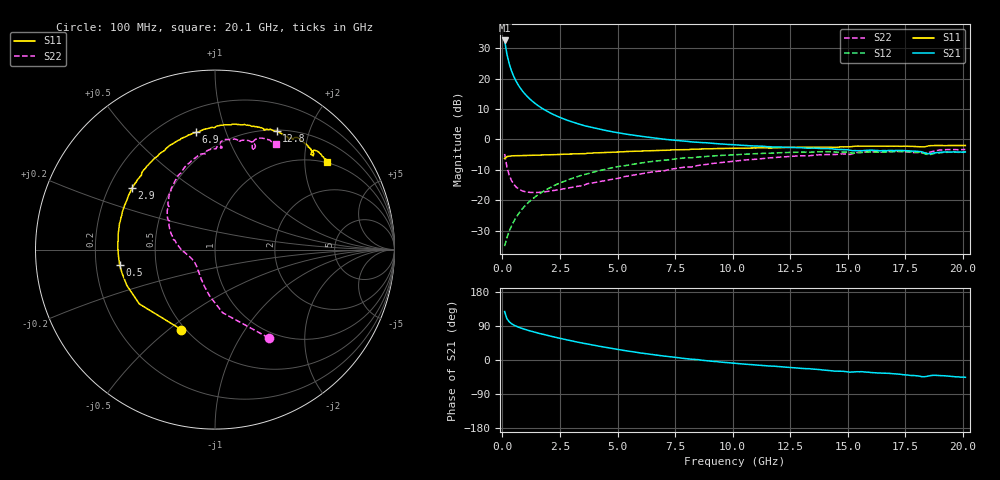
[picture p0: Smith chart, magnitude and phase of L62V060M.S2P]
!  Infineon Technologies AG
! BFR380L3 , PF131585-7, No.6, Th 09.10.01, soldered on pcb-board, measured with PP GSG850
!  Vce=2.0 V,  Ic=60.0 mA
! Common Emitter S-Parameters:  15. November 2001
#  GHz  S  MA  R  50
! f  S11  S21  S12  S22
! GHz  Mag  Ang  Mag  Ang  Mag  Ang  Mag  Ang
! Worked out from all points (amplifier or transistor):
!   201 points, 100 MHz to 20.1 GHz, reference 50 ohm
!   highest |S21| = 32.6 dB at 100 MHz (marker M1)
!   |S21| within 3 dB of that: start of sweep to 166.2 MHz
!   unconditionally stable (mu >= 1): 730.2 MHz to 4.314 GHz; 18.27 GHz to 18.57 GHz
!   at 3.4 GHz: K = 1.02, MAG = 7.5 dB, |S12| = -11.9 dB
!   at 10.1 GHz: K = 0.96, MSG = 1.6 dB, |S12| = -5.0 dB
!   at 20.1 GHz: K = 0.99, MSG = 0.0 dB, |S12| = -4.2 dB
!   S11 on the Smith chart (normalised r, x): 100 MHz: 0.48, -0.55; 500 MHz: 0.30, -0.07; 2.9 GHz: 0.30, +0.30; 6.9 GHz: 0.34, +0.79; 12.8 GHz: 0.52, +1.52; 20.1 GHz: 0.97, +2.58
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0.1  0.4834 -112.8  42.61 127.7  0.01746 57.2  0.5762 -58.6
0.2  0.519 -144.3  25.29 109.1  0.02393 58.7  0.3544 -83.1
0.3  0.5302 -157.8  17.6 100.9  0.03099 61.3  0.2588 -96.8
0.4  0.534 -165.7  13.42 95.8  0.0376 64.7  0.2098 -106.9
0.5  0.5382 -170.9  10.82 92.1  0.04477 67.0  0.1822 -114.7
0.6  0.5385 -175.0  9.05 89.3  0.05207 68.5  0.1646 -121.2
0.7  0.5399 -178.2  7.796 86.7  0.0592 69.4  0.1535 -126.7
0.8  0.541 178.9  6.84 84.4  0.06676 70.0  0.1459 -131.3
1  0.5426 174.1  5.506 80.4  0.08169 70.6  0.1375 -138.7
1.2  0.5468 169.9  4.609 76.8  0.0965 70.2  0.1343 -144.4
1.5  0.5516 164.6  3.717 71.9  0.119 69.2  0.1336 -151.0
1.8  0.5535 159.6  3.123 67.2  0.1412 67.9  0.1364 -156.3
2.9  0.5761 143.5  2.018 51.9  0.2196 60.9  0.1594 -170.7
3.5  0.583 135.3  1.711 44.3  0.2611 56.5  0.1739 -176.1
5.1  0.6197 116.9  1.27 26.8  0.361 44.4  0.231 166.8
6.8  0.6611 100.1  1.031 12.0  0.4476 32.2  0.2993 148.6
6.9  0.6619 99.2  1.021 11.1  0.451 31.4  0.2995 147.8
10.1  0.7148 75.9  0.8118 -8.7  0.5612 10.2  0.4408 120.7
12.8  0.7439 62.4  0.7318 -21.6  0.6158 -6.3  0.536 99.6
13.5  0.7458 59.0  0.7192 -24.0  0.6209 -10.2  0.5469 95.2
16.8  0.774 47.2  0.6586 -35.3  0.6242 -25.8  0.6302 75.4
20.1  0.7943 38.0  0.6238 -45.7  0.6176 -39.3  0.6827 59.9
